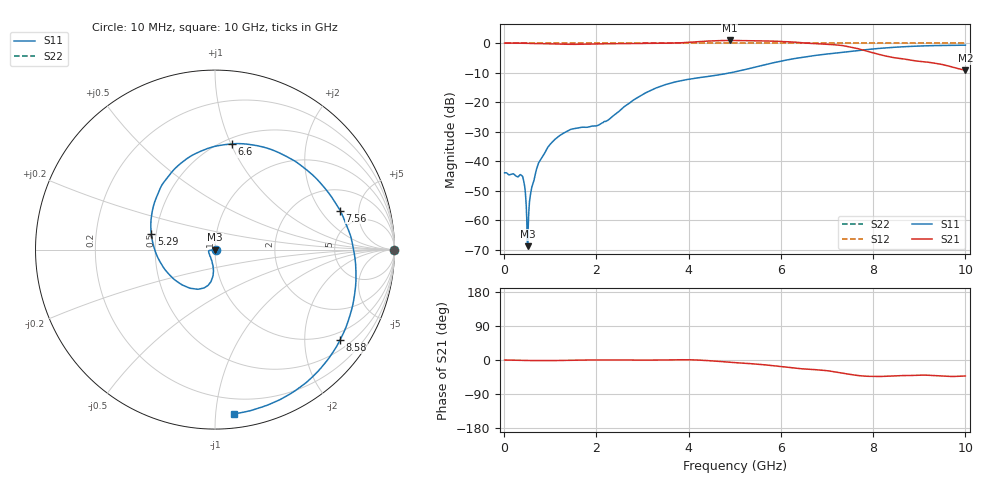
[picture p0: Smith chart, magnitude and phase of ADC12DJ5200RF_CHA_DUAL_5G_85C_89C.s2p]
! Texas Instruments, Inc.
! ADC12DJ5200RF - CH A S-Parameters (Dual Ch Mode, Fs = 5 GSPS, 85 degC case, 89 degC juntion)
! Port 1 represents the 100-ohm differenal input, Port 2 the digital output
! freq  dbS11  angS11  dbS21 angS21 dbS12 angS12 dbS22 angS22
# HZ S DB R 100
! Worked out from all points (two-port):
!   1000 points, 10 MHz to 10 GHz, reference 100 ohm
!   highest |S21| = 0.89 dB at 4.89 GHz (marker M1); lowest = -9.2 dB at 10 GHz (marker M2)
!   |S21| within 3 dB of the highest: start of sweep to 7.722 GHz
!   lowest |S11| = -68.9 dB at 510 MHz (marker M3), VSWR 1.00, Z = 100 - j0.0713 ohm
!   |S11| at or under -10 dB: start of sweep to 4.932 GHz
!   |S22| runs from 0.0 to 0.0 dB; largest |S21 - S12| = 0.78
!   S11 on the Smith chart (normalised r, x): 10 MHz: 1.01, -0.00; 5.29 GHz: 0.47, +0.10; 6.6 GHz: 0.55, +1.01; 7.56 GHz: 3.35, +3.13; 8.58 GHz: 0.75, -2.91; 10 GHz: 0.09, -1.12
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1e7  -43.98 -7.6  0.00 -0.0  0.00 0.0  0.00 0.0
3.8e8  -44.92 -10.5  -0.04 -1.1  0.00 0.0  0.00 0.0
4.3e8  -47.24 -0.5  -0.06 -1.3  0.00 0.0  0.00 0.0
4.7e8  -52.81 6.8  -0.07 -1.3  0.00 0.0  0.00 0.0
5.1e8  -68.87 -81.6  -0.09 -1.4  0.00 0.0  0.00 0.0
7.1e8  -42.37 -157.4  -0.17 -1.5  0.00 0.0  0.00 0.0
9.4e8  -35.52 -169.1  -0.23 -1.6  0.00 0.0  0.00 0.0
1.26e9  -30.80 -171.7  -0.36 -1.3  0.00 0.0  0.00 0.0
1.68e9  -28.56 -163.4  -0.40 -0.2  0.00 0.0  0.00 0.0
2.24e9  -26.25 -119.8  -0.21 0.0  0.00 0.0  0.00 0.0
3.34e9  -14.98 -96.9  -0.09 -0.2  0.00 0.0  0.00 0.0
4.19e9  -11.81 -123.4  0.47 -0.1  0.00 0.0  0.00 0.0
4.89e9  -10.14 -166.0  0.89 -5.9  0.00 0.0  0.00 0.0
5.01e9  -9.74 -174.4  0.86 -7.1  0.00 0.0  0.00 0.0
5.29e9  -8.74 165.9  0.79 -9.3  0.00 0.0  0.00 0.0
5.9e9  -6.49 126.2  0.62 -15.9  0.00 0.0  0.00 0.0
6.6e9  -4.49 81.1  -0.06 -24.3  0.00 0.0  0.00 0.0
6.67e9  -4.33 76.5  -0.15 -25.0  0.00 0.0  0.00 0.0
7.56e9  -2.73 17.4  -1.49 -39.1  0.00 0.0  0.00 0.0
8.34e9  -1.56 -25.8  -4.61 -42.6  0.00 0.0  0.00 0.0
8.58e9  -1.31 -35.9  -5.22 -41.1  0.00 0.0  0.00 0.0
1e10  -0.71 -83.2  -9.23 -42.2  0.00 0.0  0.00 0.0
